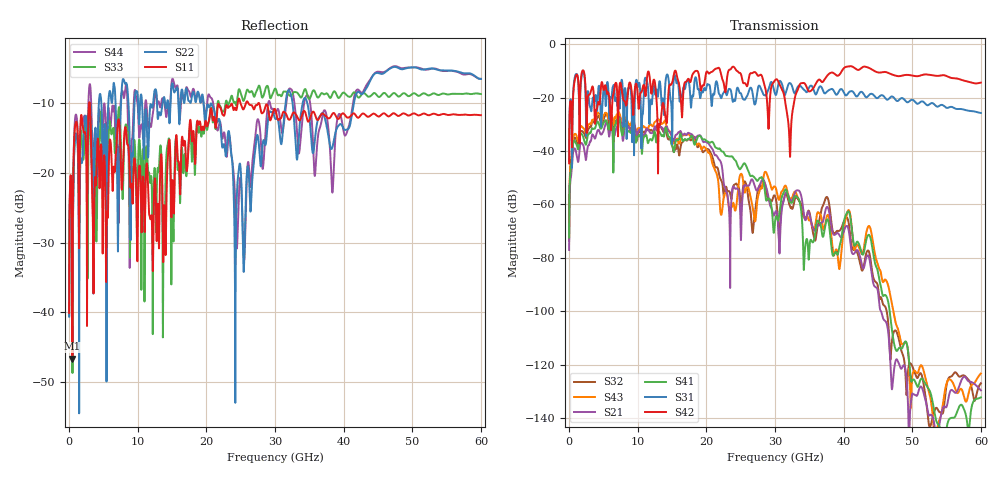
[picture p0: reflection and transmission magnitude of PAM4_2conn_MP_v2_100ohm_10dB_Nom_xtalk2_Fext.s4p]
! Info: Touchstone file created by Circ.  Input file=FAB50GbE_2conn_Midplane_Examax_Topo2_v2_100ohm_10dB_Nom.circ
# Hz S RI R 50
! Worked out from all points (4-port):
!   6000 points, 10 MHz to 60 GHz, reference 50 ohm
!   strongest paths, dB at 10 MHz, 15.01 GHz, 30.01 GHz, 45.01 GHz, 60 GHz:
!     S42: -44.6, -14.5, -13.5, -10.6, -14.4
!     S31: -43.9, -35.2, -18.6, -20.1, -25.8
!     S41: -72.4, -37.9, -66.4, -85.4, -132.3
!     S21: -77.1, -34.9, -63.1, -92.7, -129.7
!     S43: -72.0, -35.0, -53.4, -82.7, -123.3
!     S32: -73.6, -37.9, -57.0, -91.0, -127.0
!   lowest |S11| = -46.7 dB at 490 MHz (marker M1), VSWR 1.01, Z = 50.4 - j0.131 ohm
!   |S11| at or under -10 dB: start of sweep to 2.93 GHz; 3.009 GHz to 24.56 GHz (21.55 GHz wide, 156 % of centre); 27.68 GHz to end of sweep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
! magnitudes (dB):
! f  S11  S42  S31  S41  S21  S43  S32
! 10 MHz  -40.1  -44.6  -43.9  -72.4  -77.1  -72.0  -73.6
! 490 MHz  -46.7  -28.4  -27.4  -39.5  -42.9  -37.3  -39.0
! 18.96 GHz  -12.8  -12.2  -17.5  -34.4  -34.1  -37.2  -37.6
! 23.36 GHz  -10.5  -9.6  -16.8  -42.1  -64.6  -62.4  -55.1
! 32.14 GHz  -12.4  -38.1  -14.6  -59.0  -58.0  -57.7  -60.4
! 34.37 GHz  -11.2  -14.9  -17.4  -76.8  -65.7  -65.1  -65.4
! 60 GHz  -11.7  -14.4  -25.8  -132.3  -129.7  -123.3  -127.0
